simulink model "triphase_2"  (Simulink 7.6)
settings: Solver=ode15s  StartTime=0.0  StopTime=3/60  RelTol=1e-3
InitFcn:
  | clc
libraries: powerlib x6, powerlib_extras x3

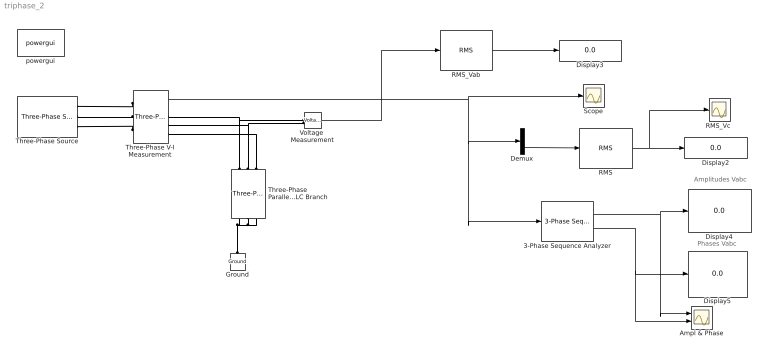
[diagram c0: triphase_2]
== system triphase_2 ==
  note: Amplitudes Vabc
  note: Phases Vabc
  3-Phase Sequence Analyzer : powerlib_extras/Measurements/3-Phase Sequence Analyzer  DialogController=POWERSYS.PowerSysDialog  SystemSampleTime=-1  f1=60  n=1  seq=Positive Negative Zero
  Ampl & Phase : Scope  NumInputPorts=2
  Demux : Demux  Outputs=3
  Display{2..5} (4 alike) : Display
  Ground : powerlib/Elements/Ground  DialogController=POWERSYS.PowerSysDialog  PhysicalDomain=powersysdomain  SubClassName=unknown  LeftPortType=p1  RightPortType=p1  LConnTagsString=a
  RMS : powerlib_extras/Measurements/RMS  DialogController=POWERSYS.PowerSysDialog  SystemSampleTime=-1  f1=60
  RMS_Vab : powerlib_extras/Measurements/RMS  DialogController=POWERSYS.PowerSysDialog  SystemSampleTime=-1  f1=60
  "RMS_Vc " : Scope
  Scope : Scope
  Three-Phase Parallel RLC Branch : powerlib/Elements/Three-Phase Parallel RLC Branch  DialogController=POWERSYS.PowerSysDialog  PhysicalDomain=powersysdomain  SubClassName=unknown  LeftPortType=p1  RightPortType=p1  LConnTagsString=A|B|C  RConnTagsString=A|B|C  BranchType=RLC  Resistance=1  Inductance=1e-3  Capacitance=1e-6  Measurements=None
  Three-Phase V-I Measurement : powerlib/Measurements/Three-Phase V-I Measurement  DialogController=POWERSYS.PowerSysDialog  SystemSampleTime=-1  VoltageMeasurement=phase-to-ground  SetLabelV=off  LabelV=Vabc  Vpu=off  VpuLL=off  CurrentMeasurement=yes  SetLabelI=off  LabelI=Iabc  Ipu=off  Pbase=100e6  Vbase=500e3  OutputType=Complex  PhasorSimulation=off  PSBequivalent=0
  Three-Phase Source : powerlib/Electrical Sources/Three-Phase Source  DialogController=POWERSYS.PowerSysDialog  SystemSampleTime=-1  Voltage=25e3  PhaseAngle=0  Frequency=60  InternalConnection=Yg  SpecifyImpedance=on  Resistance=0.8929  Inductance=16.58e-3  ShortCircuitLevel=100e6  BaseVoltage=25e3  XRratio=7
  Voltage  Measurement : powerlib/Measurements/Voltage Measurement  DialogController=POWERSYS.PowerSysDialog  SystemSampleTime=-1  PhasorSimulation=off  OutputType=Complex  PSBequivalent=0
  powergui : powerlib/powergui  Priority=1  SystemSampleTime=-1  SimulationMode=Continuous  SampleTime=50e-6  frequency=60  SPID=off  DisableSnubberDevices=off  DisableRonSwitches=off  DisableVfSwitches=off  SwTol=0  Interpol=off  frequencyindice=60  echomessages=off  HookPort=off  DisplayEquations=off  FunctionMessages=off  EnableUseOfTLC=off  x0status=blocks  RestoreLinks=warning  ResistiveCurrentMeasurement=off  Ylog=off  Xlog=on  ShowGrid=off  save=off  variable=ZData  ZoomFFT=off  StartTime=0.0  cycles=1  DisplayStyle=1  FreqAxis=off  MaxFrequency=1000  frequencyindicesteady=1  display=off  methode=off
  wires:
  Three-Phase V-I Measurement/1 -> Scope/1, Demux/1, 3-Phase Sequence Analyzer/1
  Voltage  Measurement/1 -> RMS_Vab/1
  Demux/3 -> RMS/1
  RMS/1 -> Display2/1, "RMS_Vc "/1
  RMS_Vab/1 -> Display3/1
  3-Phase Sequence Analyzer/1 -> Display4/1, Ampl & Phase/1
  3-Phase Sequence Analyzer/2 -> Display5/1, Ampl & Phase/2
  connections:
  Three-Phase Parallel RLC Branch/RConn2 -- Three-Phase Parallel RLC Branch/RConn1 -- Ground/LConn1 -- Three-Phase Parallel RLC Branch/RConn3
  Three-Phase V-I Measurement/LConn1 -- Three-Phase Source/RConn1
  Three-Phase V-I Measurement/LConn2 -- Three-Phase Source/RConn2
  Three-Phase V-I Measurement/LConn3 -- Three-Phase Source/RConn3
  Three-Phase Parallel RLC Branch/LConn1 -- Three-Phase V-I Measurement/RConn1 -- Voltage  Measurement/LConn1
  Three-Phase Parallel RLC Branch/LConn2 -- Three-Phase V-I Measurement/RConn2 -- Voltage  Measurement/LConn2
  Three-Phase Parallel RLC Branch/LConn3 -- Three-Phase V-I Measurement/RConn3
